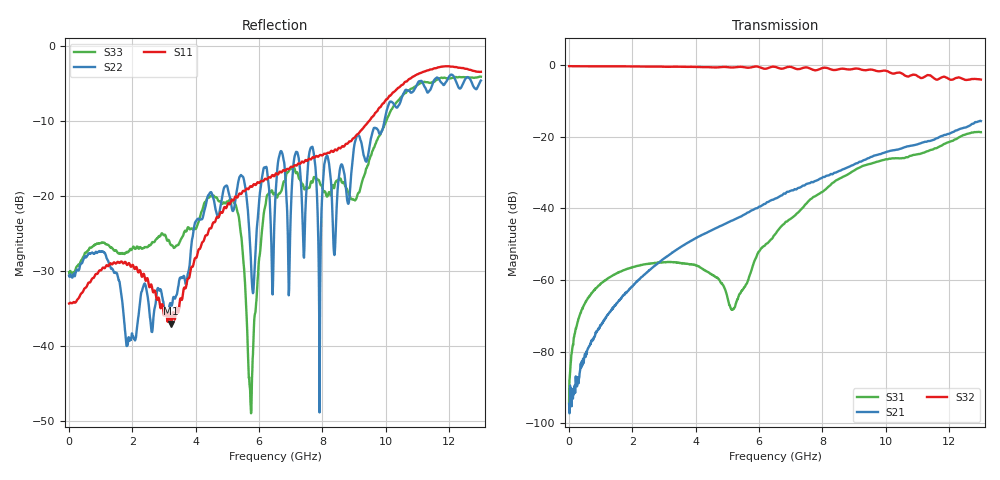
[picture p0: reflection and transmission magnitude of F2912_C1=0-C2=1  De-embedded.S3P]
! Integrated Device Technology
! Corporate Headquarters
! 6024 Silver Creek Valley Road
! San Jose, CA 95138  USA
! Phone:  1-408-284-8200
! Toll Free:  1-800-223-1366
! Webpage:  http://www.idt.com/
! Timing and RF Division
! 515 Groton Road, Suite 102
! Westford, MA 01886-6024
! Device:  F2912
! Description: High Reliability SP2T RF Switch
! Frequency:  9 kHz -  9 GHz
! Package:  4x4 mm QFN Plastic Package: 20 pin
! Ports:  3 RF, 5 DC
!  Pin  1  = GND
!  Pin  2  = GND
!  Pin  3  = RF1  =  Port 1
!  Pin  4  = GND
!  Pin  5  = GND
!  Pin  6  = GND
!  Pin  7  = GND
!  Pin  8  = RF_COM =  Port 3
!  Pin  9  = GND
!  Pin 10  = GND
!  Pin 11  = GND
!  Pin 12  = GND
!  Pin 13  = RF2  =  Port 2
!  Pin 14  = GND
!  Pin 15  = GND
!  Pin 16  = CTL2
!  Pin 17  = CTL1
!  Pin 18  = LogicCTL
!  Pin 19  = ModeCTL
!  Pin 20  = Vcc
! Logic:  3.3 V
! Mode:  2 pin control
! Voltage:  +3.30  Volts
! Current:  0.030 mA
! State:  RF2 Selected
! CTL1:  Logic LOW
! CTL2:  Logic HIGH
! Data:  The device was measured on a F2912 evaluation board which has
!  individual transmission lines to the RF pins.  Data was collected
!  using a calibrated network analyzer.  The evaluation board was
!  de-embedded using AFR (Keysight).
!  The reference plane is the edge of the package pin.
! Misc:  Action Tracker AT0438
! Date Measured:  2018-12-14
! Date:  2018-12-14  MJV
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# Hz S dB R 50
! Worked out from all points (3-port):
!   1300 points, 10 MHz to 13 GHz, reference 50 ohm
!   strongest paths, dB at 10 MHz, 3.26 GHz, 6.51 GHz, 9.76 GHz, 13 GHz:
!     S32: -0.3, -0.5, -0.5, -1.7, -4.0
!     S21: -94.7, -52.3, -37.3, -25.0, -15.6
!     S31: -94.0, -55.0, -47.3, -26.9, -18.7
!   lowest |S11| = -37.0 dB at 3.23 GHz (marker M1), VSWR 1.03, Z = 48.6 + j0.0762 ohm
!   |S11| at or under -10 dB: start of sweep to 9.481 GHz
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1e7  -34.36 178.9  -93.12 70.6  -90.69 72.7
     -94.67 56.8  -30.65 -1.5  -0.31 -0.1
     -94.01 78.2  -0.31 -0.1  -30.18 -0.7
9.9e8  -29.95 158.4  -73.07 -141.4  -61.19 80.7
       -72.62 -140.7  -27.48 46.0  -0.35 -8.1
       -61.14 80.6  -0.36 -8.1  -26.34 34.1
3.23e9  -37.05 176.8  -52.63 -168.6  -55.03 70.0
        -52.62 -168.7  -34.59 -84.3  -0.46 -26.6
        -54.99 70.2  -0.47 -26.7  -26.57 -47.3
5.23e9  -20.32 159.5  -43.21 175.9  -68.16 148.6
        -43.11 176.0  -21.34 45.4  -0.63 -43.5
        -67.69 149.4  -0.64 -44.1  -21.01 22.6
5.73e9  -18.73 168.6  -40.60 174.9  -58.23 -144.8
        -40.75 174.9  -27.15 -153.7  -0.47 -48.1
        -58.18 -147.3  -0.67 -49.4  -47.49 -43.8
6.51e9  -17.18 173.6  -37.28 170.4  -47.23 -141.1
        -37.27 170.1  -20.85 150.5  -0.66 -56.8
        -47.28 -141.9  -0.48 -56.3  -19.63 -141.5
7.67e9  -14.98 173.9  -32.95 153.9  -37.10 -147.8
        -32.64 158.9  -13.50 163.5  -0.95 -68.2
        -37.22 -147.9  -1.21 -65.7  -18.20 -109.0
7.91e9  -14.61 173.1  -31.57 157.7  -35.89 -151.4
        -31.78 156.3  -48.89 -96.9  -0.99 -70.7
        -35.90 -151.3  -1.15 -72.3  -18.15 -109.4
8.12e9  -14.42 171.4  -30.98 152.4  -34.47 -152.9
        -30.93 154.3  -14.81 118.6  -0.89 -72.6
        -34.57 -152.9  -0.76 -71.7  -19.93 -100.7
1.3e10  -3.48 118.6  -15.83 48.1  -18.73 83.7
        -15.62 50.8  -4.64 104.2  -4.25 -132.5
        -18.74 83.1  -4.04 -132.2  -4.12 149.0
